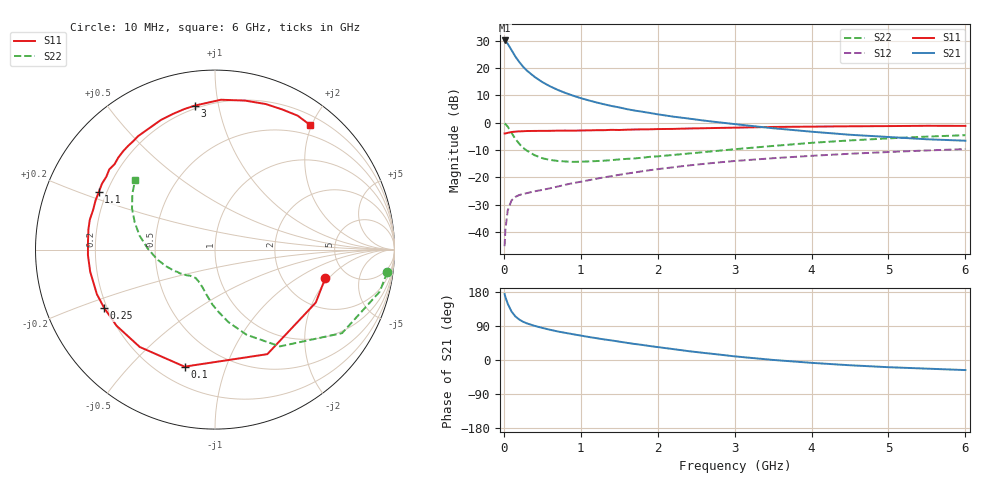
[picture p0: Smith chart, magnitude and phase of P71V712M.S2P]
! SIEMENS Small Signal Semiconductors
! BFP196
! Si NPN RF Bipolar Junction Transistor in SOT143
! VCE = 1.75 V  IC = 12 mA
! Common Emitter S-Parameters:  May  1996
# GHz  S  MA  R  50
!  f  S11  S21  S12  S22
! GHz  MAG  ANG  MAG  ANG  MAG  ANG  MAG  ANG
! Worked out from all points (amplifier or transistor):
!   36 points, 10 MHz to 6 GHz, reference 50 ohm
!   highest |S21| = 30.1 dB at 10 MHz (marker M1)
!   |S21| within 3 dB of that: start of sweep to 88.47 MHz
!   unconditionally stable (mu >= 1): 819.3 MHz to 3.346 GHz
!   at 250 MHz: K = 0.46, MSG = 23.3 dB, |S12| = -26.1 dB
!   at 1.4 GHz: K = 1.13, MAG = 10.7 dB, |S12| = -19.6 dB
!   at 6 GHz: K = 0.99, MSG = 1.5 dB, |S12| = -9.7 dB
!   S11 on the Smith chart (normalised r, x): 10 MHz: 3.45, -1.82; 100 MHz: 0.30, -0.73; 250 MHz: 0.19, -0.24; 1.1 GHz: 0.17, +0.23; 3 GHz: 0.18, +0.85; 6 GHz: 0.34, +1.97
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0.01  0.6347 -14.4  31.94 173.9  0.0055 85.2  0.9677 -7.5
0.02  0.6344 -27.7  30.83 166.3  0.0109 76.4  0.9475 -14.3
0.05  0.6515 -63.4  27.82 148.8  0.0247 63.5  0.8473 -33.3
0.1  0.6739 -104.6  21.25 127.9  0.0379 47.4  0.649 -56.2
0.15  0.6857 -127.7  16.17 115.0  0.0439 39.4  0.5056 -69.7
0.2  0.6935 -142.3  12.94 106.8  0.0474 35.6  0.4116 -79.4
0.25  0.6978 -152.3  10.58 100.9  0.0497 33.9  0.3469 -86.9
0.3  0.7035 -159.3  8.97 96.6  0.0514 34.3  0.3076 -92.5
0.4  0.7062 -170.0  6.88 90.1  0.0555 35.2  0.254 -101.0
0.5  0.7086 -177.5  5.532 84.7  0.0589 36.6  0.2236 -107.7
0.6  0.7091 176.4  4.631 79.8  0.063 38.9  0.2084 -112.9
0.7  0.7143 170.8  3.985 75.3  0.0678 40.4  0.1994 -117.2
0.9  0.7142 162.0  3.117 68.0  0.0784 43.0  0.1917 -123.9
1.1  0.7224 153.7  2.565 60.9  0.0883 44.9  0.1953 -129.3
1.3  0.729 146.1  2.176 54.4  0.0997 45.5  0.2015 -134.0
1.6  0.7439 136.4  1.768 45.3  0.1172 45.3  0.2178 -140.1
2.2  0.769 118.5  1.291 28.8  0.1526 42.1  0.2567 -152.3
3  0.8103 97.9  0.941 9.6  0.1989 34.2  0.3267 -170.4
3.5  0.8356 87.7  0.791 0.2  0.2239 28.6  0.3753 179.0
4.5  0.8589 70.8  0.601 -13.9  0.2701 17.6  0.4736 161.0
5.5  0.8769 58.3  0.497 -22.8  0.3104 6.4  0.5562 145.9
6  0.8734 52.7  0.468 -26.6  0.3288 0.3  0.5906 138.8
